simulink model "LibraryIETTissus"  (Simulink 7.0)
settings: Solver=ode45  StartTime=0.0  StopTime=10  RelTol=1e-3
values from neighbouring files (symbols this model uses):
  b = S/Sm    (= 0.1)    [Constantes.m]    (also in ConstantesBck.m)
  beta = 0.95    [Constantes.m]    (also in ResCourV1.m = 1; ResCrV1.m = 1; ResEnerV1.m = 1; ConstantesBck.m)
  C = 1    [Constantes.m]    (also in ConstantesBck.m)
  Cdl = 603E-9    (= 6.03e-07)    [Constantes.m]    (also in ResCourV1.m = 7.313e-07; ResCrV1.m = 7.313e-07; ResEnerV1.m = 7.313e-07; ConstantesBck.m)
  Cmem = 1E-6*Sm*(1-b)    (= 2.826e-08)    [Constantes.m]    (also in ConstantesBck.m = 3.14e-11; ImpedanceZtissus.m = 4e-08; Ztissus.m = 4e-08; CalculCharge.m = 1)
  Fact = 10^2    (= 100)    [Constantes.m]    (also in ConstantesBck.m)
  gk = 36    [Constantes.m]    (also in ConstantesBck.m; sim_hh.m)
  gl = 0.3    [Constantes.m]    (also in ConstantesBck.m; sim_hh.m)
  gna = 120    [Constantes.m]    (also in ConstantesBck.m; sim_hh.m)
  h0 = 0.5961    [Constantes.m]    (also in ConstantesBck.m)
  m0 = 0.0529    [Constantes.m]    (also in ConstantesBck.m)
  mK = 0    [Constantes.m]    (also in ConstantesBck.m)
  mL = 0    [Constantes.m]    (also in ConstantesBck.m)
  mNa = 0    [Constantes.m]    (also in ConstantesBck.m)
  n0 = 0.3177    [Constantes.m]    (also in ConstantesBck.m)
  rapportIE = 10    [Constantes.m]
  Rcan = 6.398E3*Sm*(1-b)    (= 180.80748)    [Constantes.m]    (also in ConstantesBck.m = 0.03454; ImpedanceZtissus.m = 44; Ztissus.m = 44)
  Rct = 185.6E3    (= 185600)    [Constantes.m]    (also in ResCourV1.m = 605200; ResCrV1.m = 605200; ResEnerV1.m = 605200; ConstantesBck.m)
  Rext = 2.9E3    (= 2900)    [Constantes.m]    (also in ConstantesBck.m)
  Rint = 2.9E2    (= 290)    [Constantes.m]    (also in ConstantesBck.m = 400)
  sigma = 66466    [Constantes.m]    (also in ResCourV1.m = 68000; ResCrV1.m = 68000; ResEnerV1.m = 68000; ConstantesBck.m)
  Sm = 3.14e-2    (= 0.0314)    [Constantes.m]    (also in ConstantesBck.m = 0.000314)
  Vk = -82    [Constantes.m]    (also in ConstantesBck.m)
  Vl = -59    [Constantes.m]    (also in ConstantesBck.m)
  Vna = 45    [Constantes.m]    (also in ConstantesBck.m)
  Vr = -70    [Constantes.m]    (also in ConstantesBck.m)
undefined symbols (not defined in the file or in its folder): ln
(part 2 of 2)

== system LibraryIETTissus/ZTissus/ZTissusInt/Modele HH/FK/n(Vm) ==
  note: V
  note: alpha_*(1-n)
  note: beta_n*n
  note: n
  note: n
  Vm : Inport  OutDataType=sfix(16)  OutScaling=2^0
  (1-n) : Fcn  Expr=1-u
  Integrator1 : Integrator  InitialCondition=n0
  Product : Product  OutDataType=sfix(16)  OutScaling=2^0
  Product1 : Product  OutDataType=sfix(16)  OutScaling=2^0
  Sum1 : Sum  Inputs=+-  OutDataType=sfix(16)  OutScaling=2^0
  V : Fcn  Expr=u-Vr
  alpha_n : Fcn  Expr=(0.01*(10-u))/(exp((10-u)/10)-1)
  beta_n : Fcn  Expr=0.125*exp(-u/80)
  n : Outport  OutDataType=sfix(16)  OutScaling=2^0  InitialOutput=0
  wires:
  V/1 -> alpha_n/1, beta_n/1
  alpha_n/1 -> Product/2
  (1-n)/1 -> Product/1
  beta_n/1 -> Product1/1
  Product/1 -> Sum1/1
  Product1/1 -> Sum1/2
  Sum1/1 -> Integrator1/1
  Integrator1/1 -> (1-n)/1, Product1/2, n/1
  Vm/1 -> V/1

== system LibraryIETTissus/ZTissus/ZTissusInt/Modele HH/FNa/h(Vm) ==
  note: h
  note: h
  note: beta_h*h
  note: alpha_h*(1-h)
  note: V
  Vm : Inport  OutDataType=sfix(16)  OutScaling=2^0
  (1-h) : Fcn  Expr=1-u
  Integrator1 : Integrator  InitialCondition=h0
  Product : Product  OutDataType=sfix(16)  OutScaling=2^0
  Product1 : Product  OutDataType=sfix(16)  OutScaling=2^0
  Sum1 : Sum  Inputs=+-  OutDataType=sfix(16)  OutScaling=2^0
  V : Fcn  Expr=u-Vr
  alpha_h : Fcn  Expr=0.07*exp(-u/20)
  beta_h : Fcn  Expr=1/(exp((30-u)/10)+1)
  h : Outport  OutDataType=sfix(16)  OutScaling=2^0  InitialOutput=0
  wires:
  Vm/1 -> V/1
  Integrator1/1 -> h/1, Product1/2, (1-h)/1
  Sum1/1 -> Integrator1/1
  Product1/1 -> Sum1/2
  Product/1 -> Sum1/1
  beta_h/1 -> Product1/1
  (1-h)/1 -> Product/1
  alpha_h/1 -> Product/2
  V/1 -> beta_h/1, alpha_h/1

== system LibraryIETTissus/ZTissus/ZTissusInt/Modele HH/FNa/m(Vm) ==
  note: m
  note: m
  note: beta_m*m
  note: alpha_m*(1-m)
  note: V
  Vm : Inport  OutDataType=sfix(16)  OutScaling=2^0
  (1-m) : Fcn  Expr=1-u
  Integrator1 : Integrator  InitialCondition=m0
  Product : Product  OutDataType=sfix(16)  OutScaling=2^0
  Product1 : Product  OutDataType=sfix(16)  OutScaling=2^0
  Sum1 : Sum  Inputs=+-  OutDataType=sfix(16)  OutScaling=2^0
  V : Fcn  Expr=u-Vr
  alpha_m : Fcn  Expr=(0.1*(25-u))/(exp((25-u)/10)-1)
  beta_m : Fcn  Expr=4*exp(-u/18)
  n : Outport  OutDataType=sfix(16)  OutScaling=2^0  InitialOutput=0
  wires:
  Vm/1 -> V/1
  Integrator1/1 -> n/1, Product1/2, (1-m)/1
  Sum1/1 -> Integrator1/1
  Product1/1 -> Sum1/2
  Product/1 -> Sum1/1
  beta_m/1 -> Product1/1
  (1-m)/1 -> Product/1
  alpha_m/1 -> Product/2
  V/1 -> beta_m/1, alpha_m/1

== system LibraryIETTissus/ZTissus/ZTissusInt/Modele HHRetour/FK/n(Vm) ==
  note: V
  note: alpha_*(1-n)
  note: beta_n*n
  note: n
  note: n
  Vm : Inport  OutDataType=sfix(16)  OutScaling=2^0
  (1-n) : Fcn  Expr=1-u
  Integrator1 : Integrator  InitialCondition=n0
  Product : Product  OutDataType=sfix(16)  OutScaling=2^0
  Product1 : Product  OutDataType=sfix(16)  OutScaling=2^0
  Sum1 : Sum  Inputs=+-  OutDataType=sfix(16)  OutScaling=2^0
  V : Fcn  Expr=u-Vr
  alpha_n : Fcn  Expr=(0.01*(10-u))/(exp((10-u)/10)-1)
  beta_n : Fcn  Expr=0.125*exp(-u/80)
  n : Outport  OutDataType=sfix(16)  OutScaling=2^0  InitialOutput=0
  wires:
  V/1 -> alpha_n/1, beta_n/1
  alpha_n/1 -> Product/2
  (1-n)/1 -> Product/1
  beta_n/1 -> Product1/1
  Product/1 -> Sum1/1
  Product1/1 -> Sum1/2
  Sum1/1 -> Integrator1/1
  Integrator1/1 -> (1-n)/1, Product1/2, n/1
  Vm/1 -> V/1

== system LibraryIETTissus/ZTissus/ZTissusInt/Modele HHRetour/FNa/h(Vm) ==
  note: h
  note: h
  note: beta_h*h
  note: alpha_h*(1-h)
  note: V
  Vm : Inport  OutDataType=sfix(16)  OutScaling=2^0
  (1-h) : Fcn  Expr=1-u
  Integrator1 : Integrator  InitialCondition=h0
  Product : Product  OutDataType=sfix(16)  OutScaling=2^0
  Product1 : Product  OutDataType=sfix(16)  OutScaling=2^0
  Sum1 : Sum  Inputs=+-  OutDataType=sfix(16)  OutScaling=2^0
  V : Fcn  Expr=u-Vr
  alpha_h : Fcn  Expr=0.07*exp(-u/20)
  beta_h : Fcn  Expr=1/(exp((30-u)/10)+1)
  h : Outport  OutDataType=sfix(16)  OutScaling=2^0  InitialOutput=0
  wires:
  Vm/1 -> V/1
  Integrator1/1 -> h/1, Product1/2, (1-h)/1
  Sum1/1 -> Integrator1/1
  Product1/1 -> Sum1/2
  Product/1 -> Sum1/1
  beta_h/1 -> Product1/1
  (1-h)/1 -> Product/1
  alpha_h/1 -> Product/2
  V/1 -> beta_h/1, alpha_h/1

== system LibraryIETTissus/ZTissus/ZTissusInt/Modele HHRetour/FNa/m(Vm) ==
  note: m
  note: m
  note: beta_m*m
  note: alpha_m*(1-m)
  note: V
  Vm : Inport  OutDataType=sfix(16)  OutScaling=2^0
  (1-m) : Fcn  Expr=1-u
  Integrator1 : Integrator  InitialCondition=m0
  Product : Product  OutDataType=sfix(16)  OutScaling=2^0
  Product1 : Product  OutDataType=sfix(16)  OutScaling=2^0
  Sum1 : Sum  Inputs=+-  OutDataType=sfix(16)  OutScaling=2^0
  V : Fcn  Expr=u-Vr
  alpha_m : Fcn  Expr=(0.1*(25-u))/(exp((25-u)/10)-1)
  beta_m : Fcn  Expr=4*exp(-u/18)
  n : Outport  OutDataType=sfix(16)  OutScaling=2^0  InitialOutput=0
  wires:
  Vm/1 -> V/1
  Integrator1/1 -> n/1, Product1/2, (1-m)/1
  Sum1/1 -> Integrator1/1
  Product1/1 -> Sum1/2
  Product/1 -> Sum1/1
  beta_m/1 -> Product1/1
  (1-m)/1 -> Product/1
  alpha_m/1 -> Product/2
  V/1 -> beta_m/1, alpha_m/1

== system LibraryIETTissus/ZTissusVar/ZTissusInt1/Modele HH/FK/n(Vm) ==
  note: V
  note: alpha_*(1-n)
  note: beta_n*n
  note: n
  note: n
  Vm : Inport  OutDataType=sfix(16)  OutScaling=2^0
  (1-n) : Fcn  Expr=1-u
  Integrator1 : Integrator  InitialCondition=n0
  Product : Product  OutDataType=sfix(16)  OutScaling=2^0
  Product1 : Product  OutDataType=sfix(16)  OutScaling=2^0
  Sum1 : Sum  Inputs=+-  OutDataType=sfix(16)  OutScaling=2^0
  V : Fcn  Expr=u-Vr
  alpha_n : Fcn  Expr=(0.01*(10-u))/(exp((10-u)/10)-1)
  beta_n : Fcn  Expr=0.125*exp(-u/80)
  n : Outport  OutDataType=sfix(16)  OutScaling=2^0  InitialOutput=0
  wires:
  V/1 -> alpha_n/1, beta_n/1
  alpha_n/1 -> Product/2
  (1-n)/1 -> Product/1
  beta_n/1 -> Product1/1
  Product/1 -> Sum1/1
  Product1/1 -> Sum1/2
  Sum1/1 -> Integrator1/1
  Integrator1/1 -> (1-n)/1, Product1/2, n/1
  Vm/1 -> V/1

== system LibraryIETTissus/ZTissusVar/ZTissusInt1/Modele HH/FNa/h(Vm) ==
  note: h
  note: h
  note: beta_h*h
  note: alpha_h*(1-h)
  note: V
  Vm : Inport  OutDataType=sfix(16)  OutScaling=2^0
  (1-h) : Fcn  Expr=1-u
  Integrator1 : Integrator  InitialCondition=h0
  Product : Product  OutDataType=sfix(16)  OutScaling=2^0
  Product1 : Product  OutDataType=sfix(16)  OutScaling=2^0
  Sum1 : Sum  Inputs=+-  OutDataType=sfix(16)  OutScaling=2^0
  V : Fcn  Expr=u-Vr
  alpha_h : Fcn  Expr=0.07*exp(-u/20)
  beta_h : Fcn  Expr=1/(exp((30-u)/10)+1)
  h : Outport  OutDataType=sfix(16)  OutScaling=2^0  InitialOutput=0
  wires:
  Vm/1 -> V/1
  Integrator1/1 -> h/1, Product1/2, (1-h)/1
  Sum1/1 -> Integrator1/1
  Product1/1 -> Sum1/2
  Product/1 -> Sum1/1
  beta_h/1 -> Product1/1
  (1-h)/1 -> Product/1
  alpha_h/1 -> Product/2
  V/1 -> beta_h/1, alpha_h/1

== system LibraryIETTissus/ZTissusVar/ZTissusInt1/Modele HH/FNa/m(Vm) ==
  note: m
  note: m
  note: beta_m*m
  note: alpha_m*(1-m)
  note: V
  Vm : Inport  OutDataType=sfix(16)  OutScaling=2^0
  (1-m) : Fcn  Expr=1-u
  Integrator1 : Integrator  InitialCondition=m0
  Product : Product  OutDataType=sfix(16)  OutScaling=2^0
  Product1 : Product  OutDataType=sfix(16)  OutScaling=2^0
  Sum1 : Sum  Inputs=+-  OutDataType=sfix(16)  OutScaling=2^0
  V : Fcn  Expr=u-Vr
  alpha_m : Fcn  Expr=(0.1*(25-u))/(exp((25-u)/10)-1)
  beta_m : Fcn  Expr=4*exp(-u/18)
  n : Outport  OutDataType=sfix(16)  OutScaling=2^0  InitialOutput=0
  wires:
  Vm/1 -> V/1
  Integrator1/1 -> n/1, Product1/2, (1-m)/1
  Sum1/1 -> Integrator1/1
  Product1/1 -> Sum1/2
  Product/1 -> Sum1/1
  beta_m/1 -> Product1/1
  (1-m)/1 -> Product/1
  alpha_m/1 -> Product/2
  V/1 -> beta_m/1, alpha_m/1

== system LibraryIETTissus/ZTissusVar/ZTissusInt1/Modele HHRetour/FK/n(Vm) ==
  note: V
  note: alpha_*(1-n)
  note: beta_n*n
  note: n
  note: n
  Vm : Inport  OutDataType=sfix(16)  OutScaling=2^0
  (1-n) : Fcn  Expr=1-u
  Integrator1 : Integrator  InitialCondition=n0
  Product : Product  OutDataType=sfix(16)  OutScaling=2^0
  Product1 : Product  OutDataType=sfix(16)  OutScaling=2^0
  Sum1 : Sum  Inputs=+-  OutDataType=sfix(16)  OutScaling=2^0
  V : Fcn  Expr=u-Vr
  alpha_n : Fcn  Expr=(0.01*(10-u))/(exp((10-u)/10)-1)
  beta_n : Fcn  Expr=0.125*exp(-u/80)
  n : Outport  OutDataType=sfix(16)  OutScaling=2^0  InitialOutput=0
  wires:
  V/1 -> alpha_n/1, beta_n/1
  alpha_n/1 -> Product/2
  (1-n)/1 -> Product/1
  beta_n/1 -> Product1/1
  Product/1 -> Sum1/1
  Product1/1 -> Sum1/2
  Sum1/1 -> Integrator1/1
  Integrator1/1 -> (1-n)/1, Product1/2, n/1
  Vm/1 -> V/1

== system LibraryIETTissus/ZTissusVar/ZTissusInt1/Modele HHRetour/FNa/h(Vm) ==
  note: h
  note: h
  note: beta_h*h
  note: alpha_h*(1-h)
  note: V
  Vm : Inport  OutDataType=sfix(16)  OutScaling=2^0
  (1-h) : Fcn  Expr=1-u
  Integrator1 : Integrator  InitialCondition=h0
  Product : Product  OutDataType=sfix(16)  OutScaling=2^0
  Product1 : Product  OutDataType=sfix(16)  OutScaling=2^0
  Sum1 : Sum  Inputs=+-  OutDataType=sfix(16)  OutScaling=2^0
  V : Fcn  Expr=u-Vr
  alpha_h : Fcn  Expr=0.07*exp(-u/20)
  beta_h : Fcn  Expr=1/(exp((30-u)/10)+1)
  h : Outport  OutDataType=sfix(16)  OutScaling=2^0  InitialOutput=0
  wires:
  Vm/1 -> V/1
  Integrator1/1 -> h/1, Product1/2, (1-h)/1
  Sum1/1 -> Integrator1/1
  Product1/1 -> Sum1/2
  Product/1 -> Sum1/1
  beta_h/1 -> Product1/1
  (1-h)/1 -> Product/1
  alpha_h/1 -> Product/2
  V/1 -> beta_h/1, alpha_h/1

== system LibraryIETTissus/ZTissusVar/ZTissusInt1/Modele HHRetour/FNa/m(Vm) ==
  note: m
  note: m
  note: beta_m*m
  note: alpha_m*(1-m)
  note: V
  Vm : Inport  OutDataType=sfix(16)  OutScaling=2^0
  (1-m) : Fcn  Expr=1-u
  Integrator1 : Integrator  InitialCondition=m0
  Product : Product  OutDataType=sfix(16)  OutScaling=2^0
  Product1 : Product  OutDataType=sfix(16)  OutScaling=2^0
  Sum1 : Sum  Inputs=+-  OutDataType=sfix(16)  OutScaling=2^0
  V : Fcn  Expr=u-Vr
  alpha_m : Fcn  Expr=(0.1*(25-u))/(exp((25-u)/10)-1)
  beta_m : Fcn  Expr=4*exp(-u/18)
  n : Outport  OutDataType=sfix(16)  OutScaling=2^0  InitialOutput=0
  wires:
  Vm/1 -> V/1
  Integrator1/1 -> n/1, Product1/2, (1-m)/1
  Sum1/1 -> Integrator1/1
  Product1/1 -> Sum1/2
  Product/1 -> Sum1/1
  beta_m/1 -> Product1/1
  (1-m)/1 -> Product/1
  alpha_m/1 -> Product/2
  V/1 -> beta_m/1, alpha_m/1

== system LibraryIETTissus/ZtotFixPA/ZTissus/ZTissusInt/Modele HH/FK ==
  note: gkm
  note: (Vm-Vk0)
  FKIn : Inport  OutDataType=sfix(16)  OutScaling=2^0
  (Vm-Vk0) : Fcn  Expr=(u-Vk)
  Product : Product  OutDataType=sfix(16)  OutScaling=2^0
  n(Vm) : Subsystem
  n^4 : Fcn  Expr=gk*(u^4)
  FKout : Outport  OutDataType=sfix(16)  OutScaling=2^0  InitialOutput=0
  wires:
  n(Vm)/1(n) -> n^4/1
  (Vm-Vk0)/1 -> Product/2
  Product/1 -> FKout/1
  n^4/1 -> Product/1
  FKIn/1 -> n(Vm)/1(Vm), (Vm-Vk0)/1

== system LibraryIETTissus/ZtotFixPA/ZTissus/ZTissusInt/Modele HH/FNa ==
  note: gNa*m^3
  note: m
  note: h
  note: gNam
  note: (Vm-VNa0)
  FNaIn : Inport  OutDataType=sfix(16)  OutScaling=2^0
  (Vm-VNa0) : Fcn  Expr=(u-Vna)
  Product : Product  OutDataType=sfix(16)  OutScaling=2^0
  Product1 : Product  OutDataType=sfix(16)  OutScaling=2^0
  gna*m^3 : Fcn  Expr=gna*u^3
  h(Vm) : Subsystem
  m(Vm) : Subsystem
  FNaOut : Outport  OutDataType=sfix(16)  OutScaling=2^0  InitialOutput=0
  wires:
  (Vm-VNa0)/1 -> Product1/2
  gna*m^3/1 -> Product/1
  Product1/1 -> FNaOut/1
  FNaIn/1 -> m(Vm)/1(Vm), h(Vm)/1(Vm), (Vm-VNa0)/1
  m(Vm)/1(n) -> gna*m^3/1
  h(Vm)/1(h) -> Product/2
  Product/1 -> Product1/1

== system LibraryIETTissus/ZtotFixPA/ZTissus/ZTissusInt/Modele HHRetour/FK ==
  note: gkm
  note: (Vm-Vk0)
  FKIn : Inport  OutDataType=sfix(16)  OutScaling=2^0
  (Vm-Vk0) : Fcn  Expr=(u-Vk)
  Product : Product  OutDataType=sfix(16)  OutScaling=2^0
  n(Vm) : Subsystem
  n^4 : Fcn  Expr=gk*(u^4)
  FKout : Outport  OutDataType=sfix(16)  OutScaling=2^0  InitialOutput=0
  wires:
  n(Vm)/1(n) -> n^4/1
  (Vm-Vk0)/1 -> Product/2
  Product/1 -> FKout/1
  n^4/1 -> Product/1
  FKIn/1 -> n(Vm)/1(Vm), (Vm-Vk0)/1

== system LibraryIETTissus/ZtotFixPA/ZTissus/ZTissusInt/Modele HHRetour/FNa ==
  note: gNa*m^3
  note: m
  note: h
  note: gNam
  note: (Vm-VNa0)
  FNaIn : Inport  OutDataType=sfix(16)  OutScaling=2^0
  (Vm-VNa0) : Fcn  Expr=(u-Vna)
  Product : Product  OutDataType=sfix(16)  OutScaling=2^0
  Product1 : Product  OutDataType=sfix(16)  OutScaling=2^0
  gna*m^3 : Fcn  Expr=gna*u^3
  h(Vm) : Subsystem
  m(Vm) : Subsystem
  FNaOut : Outport  OutDataType=sfix(16)  OutScaling=2^0  InitialOutput=0
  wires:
  (Vm-VNa0)/1 -> Product1/2
  gna*m^3/1 -> Product/1
  Product1/1 -> FNaOut/1
  FNaIn/1 -> m(Vm)/1(Vm), h(Vm)/1(Vm), (Vm-VNa0)/1
  m(Vm)/1(n) -> gna*m^3/1
  h(Vm)/1(h) -> Product/2
  Product/1 -> Product1/1

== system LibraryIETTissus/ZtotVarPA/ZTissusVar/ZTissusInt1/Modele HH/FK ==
  note: gkm
  note: (Vm-Vk0)
  FKIn : Inport  OutDataType=sfix(16)  OutScaling=2^0
  (Vm-Vk0) : Fcn  Expr=(u-Vk)
  Product : Product  OutDataType=sfix(16)  OutScaling=2^0
  n(Vm) : Subsystem
  n^4 : Fcn  Expr=gk*(u^4)
  FKout : Outport  OutDataType=sfix(16)  OutScaling=2^0  InitialOutput=0
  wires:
  n(Vm)/1(n) -> n^4/1
  (Vm-Vk0)/1 -> Product/2
  Product/1 -> FKout/1
  n^4/1 -> Product/1
  FKIn/1 -> n(Vm)/1(Vm), (Vm-Vk0)/1

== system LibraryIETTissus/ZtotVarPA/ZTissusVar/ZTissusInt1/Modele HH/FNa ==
  note: gNa*m^3
  note: m
  note: h
  note: gNam
  note: (Vm-VNa0)
  FNaIn : Inport  OutDataType=sfix(16)  OutScaling=2^0
  (Vm-VNa0) : Fcn  Expr=(u-Vna)
  Product : Product  OutDataType=sfix(16)  OutScaling=2^0
  Product1 : Product  OutDataType=sfix(16)  OutScaling=2^0
  gna*m^3 : Fcn  Expr=gna*u^3
  h(Vm) : Subsystem
  m(Vm) : Subsystem
  FNaOut : Outport  OutDataType=sfix(16)  OutScaling=2^0  InitialOutput=0
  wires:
  (Vm-VNa0)/1 -> Product1/2
  gna*m^3/1 -> Product/1
  Product1/1 -> FNaOut/1
  FNaIn/1 -> m(Vm)/1(Vm), h(Vm)/1(Vm), (Vm-VNa0)/1
  m(Vm)/1(n) -> gna*m^3/1
  h(Vm)/1(h) -> Product/2
  Product/1 -> Product1/1

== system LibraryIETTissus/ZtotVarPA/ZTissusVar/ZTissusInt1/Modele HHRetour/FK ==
  note: gkm
  note: (Vm-Vk0)
  FKIn : Inport  OutDataType=sfix(16)  OutScaling=2^0
  (Vm-Vk0) : Fcn  Expr=(u-Vk)
  Product : Product  OutDataType=sfix(16)  OutScaling=2^0
  n(Vm) : Subsystem
  n^4 : Fcn  Expr=gk*(u^4)
  FKout : Outport  OutDataType=sfix(16)  OutScaling=2^0  InitialOutput=0
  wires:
  n(Vm)/1(n) -> n^4/1
  (Vm-Vk0)/1 -> Product/2
  Product/1 -> FKout/1
  n^4/1 -> Product/1
  FKIn/1 -> n(Vm)/1(Vm), (Vm-Vk0)/1

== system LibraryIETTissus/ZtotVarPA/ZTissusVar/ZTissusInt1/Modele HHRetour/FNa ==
  note: gNa*m^3
  note: m
  note: h
  note: gNam
  note: (Vm-VNa0)
  FNaIn : Inport  OutDataType=sfix(16)  OutScaling=2^0
  (Vm-VNa0) : Fcn  Expr=(u-Vna)
  Product : Product  OutDataType=sfix(16)  OutScaling=2^0
  Product1 : Product  OutDataType=sfix(16)  OutScaling=2^0
  gna*m^3 : Fcn  Expr=gna*u^3
  h(Vm) : Subsystem
  m(Vm) : Subsystem
  FNaOut : Outport  OutDataType=sfix(16)  OutScaling=2^0  InitialOutput=0
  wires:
  (Vm-VNa0)/1 -> Product1/2
  gna*m^3/1 -> Product/1
  Product1/1 -> FNaOut/1
  FNaIn/1 -> m(Vm)/1(Vm), h(Vm)/1(Vm), (Vm-VNa0)/1
  m(Vm)/1(n) -> gna*m^3/1
  h(Vm)/1(h) -> Product/2
  Product/1 -> Product1/1

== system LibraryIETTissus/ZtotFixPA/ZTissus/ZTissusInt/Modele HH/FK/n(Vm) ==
  note: V
  note: alpha_*(1-n)
  note: beta_n*n
  note: n
  note: n
  Vm : Inport  OutDataType=sfix(16)  OutScaling=2^0
  (1-n) : Fcn  Expr=1-u
  Integrator1 : Integrator  InitialCondition=n0
  Product : Product  OutDataType=sfix(16)  OutScaling=2^0
  Product1 : Product  OutDataType=sfix(16)  OutScaling=2^0
  Sum1 : Sum  Inputs=+-  OutDataType=sfix(16)  OutScaling=2^0
  V : Fcn  Expr=u-Vr
  alpha_n : Fcn  Expr=(0.01*(10-u))/(exp((10-u)/10)-1)
  beta_n : Fcn  Expr=0.125*exp(-u/80)
  n : Outport  OutDataType=sfix(16)  OutScaling=2^0  InitialOutput=0
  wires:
  V/1 -> alpha_n/1, beta_n/1
  alpha_n/1 -> Product/2
  (1-n)/1 -> Product/1
  beta_n/1 -> Product1/1
  Product/1 -> Sum1/1
  Product1/1 -> Sum1/2
  Sum1/1 -> Integrator1/1
  Integrator1/1 -> (1-n)/1, Product1/2, n/1
  Vm/1 -> V/1

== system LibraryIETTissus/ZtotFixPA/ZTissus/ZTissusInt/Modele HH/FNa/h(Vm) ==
  note: h
  note: h
  note: beta_h*h
  note: alpha_h*(1-h)
  note: V
  Vm : Inport  OutDataType=sfix(16)  OutScaling=2^0
  (1-h) : Fcn  Expr=1-u
  Integrator1 : Integrator  InitialCondition=h0
  Product : Product  OutDataType=sfix(16)  OutScaling=2^0
  Product1 : Product  OutDataType=sfix(16)  OutScaling=2^0
  Sum1 : Sum  Inputs=+-  OutDataType=sfix(16)  OutScaling=2^0
  V : Fcn  Expr=u-Vr
  alpha_h : Fcn  Expr=0.07*exp(-u/20)
  beta_h : Fcn  Expr=1/(exp((30-u)/10)+1)
  h : Outport  OutDataType=sfix(16)  OutScaling=2^0  InitialOutput=0
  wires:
  Vm/1 -> V/1
  Integrator1/1 -> h/1, Product1/2, (1-h)/1
  Sum1/1 -> Integrator1/1
  Product1/1 -> Sum1/2
  Product/1 -> Sum1/1
  beta_h/1 -> Product1/1
  (1-h)/1 -> Product/1
  alpha_h/1 -> Product/2
  V/1 -> beta_h/1, alpha_h/1

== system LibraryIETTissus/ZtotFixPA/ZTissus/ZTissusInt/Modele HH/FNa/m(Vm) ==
  note: m
  note: m
  note: beta_m*m
  note: alpha_m*(1-m)
  note: V
  Vm : Inport  OutDataType=sfix(16)  OutScaling=2^0
  (1-m) : Fcn  Expr=1-u
  Integrator1 : Integrator  InitialCondition=m0
  Product : Product  OutDataType=sfix(16)  OutScaling=2^0
  Product1 : Product  OutDataType=sfix(16)  OutScaling=2^0
  Sum1 : Sum  Inputs=+-  OutDataType=sfix(16)  OutScaling=2^0
  V : Fcn  Expr=u-Vr
  alpha_m : Fcn  Expr=(0.1*(25-u))/(exp((25-u)/10)-1)
  beta_m : Fcn  Expr=4*exp(-u/18)
  n : Outport  OutDataType=sfix(16)  OutScaling=2^0  InitialOutput=0
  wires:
  Vm/1 -> V/1
  Integrator1/1 -> n/1, Product1/2, (1-m)/1
  Sum1/1 -> Integrator1/1
  Product1/1 -> Sum1/2
  Product/1 -> Sum1/1
  beta_m/1 -> Product1/1
  (1-m)/1 -> Product/1
  alpha_m/1 -> Product/2
  V/1 -> beta_m/1, alpha_m/1

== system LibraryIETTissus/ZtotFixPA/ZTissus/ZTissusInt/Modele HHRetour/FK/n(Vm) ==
  note: V
  note: alpha_*(1-n)
  note: beta_n*n
  note: n
  note: n
  Vm : Inport  OutDataType=sfix(16)  OutScaling=2^0
  (1-n) : Fcn  Expr=1-u
  Integrator1 : Integrator  InitialCondition=n0
  Product : Product  OutDataType=sfix(16)  OutScaling=2^0
  Product1 : Product  OutDataType=sfix(16)  OutScaling=2^0
  Sum1 : Sum  Inputs=+-  OutDataType=sfix(16)  OutScaling=2^0
  V : Fcn  Expr=u-Vr
  alpha_n : Fcn  Expr=(0.01*(10-u))/(exp((10-u)/10)-1)
  beta_n : Fcn  Expr=0.125*exp(-u/80)
  n : Outport  OutDataType=sfix(16)  OutScaling=2^0  InitialOutput=0
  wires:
  V/1 -> alpha_n/1, beta_n/1
  alpha_n/1 -> Product/2
  (1-n)/1 -> Product/1
  beta_n/1 -> Product1/1
  Product/1 -> Sum1/1
  Product1/1 -> Sum1/2
  Sum1/1 -> Integrator1/1
  Integrator1/1 -> (1-n)/1, Product1/2, n/1
  Vm/1 -> V/1

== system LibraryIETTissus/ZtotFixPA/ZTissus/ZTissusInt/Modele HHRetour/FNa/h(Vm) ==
  note: h
  note: h
  note: beta_h*h
  note: alpha_h*(1-h)
  note: V
  Vm : Inport  OutDataType=sfix(16)  OutScaling=2^0
  (1-h) : Fcn  Expr=1-u
  Integrator1 : Integrator  InitialCondition=h0
  Product : Product  OutDataType=sfix(16)  OutScaling=2^0
  Product1 : Product  OutDataType=sfix(16)  OutScaling=2^0
  Sum1 : Sum  Inputs=+-  OutDataType=sfix(16)  OutScaling=2^0
  V : Fcn  Expr=u-Vr
  alpha_h : Fcn  Expr=0.07*exp(-u/20)
  beta_h : Fcn  Expr=1/(exp((30-u)/10)+1)
  h : Outport  OutDataType=sfix(16)  OutScaling=2^0  InitialOutput=0
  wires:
  Vm/1 -> V/1
  Integrator1/1 -> h/1, Product1/2, (1-h)/1
  Sum1/1 -> Integrator1/1
  Product1/1 -> Sum1/2
  Product/1 -> Sum1/1
  beta_h/1 -> Product1/1
  (1-h)/1 -> Product/1
  alpha_h/1 -> Product/2
  V/1 -> beta_h/1, alpha_h/1

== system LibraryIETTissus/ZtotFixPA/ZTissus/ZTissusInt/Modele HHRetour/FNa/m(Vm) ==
  note: m
  note: m
  note: beta_m*m
  note: alpha_m*(1-m)
  note: V
  Vm : Inport  OutDataType=sfix(16)  OutScaling=2^0
  (1-m) : Fcn  Expr=1-u
  Integrator1 : Integrator  InitialCondition=m0
  Product : Product  OutDataType=sfix(16)  OutScaling=2^0
  Product1 : Product  OutDataType=sfix(16)  OutScaling=2^0
  Sum1 : Sum  Inputs=+-  OutDataType=sfix(16)  OutScaling=2^0
  V : Fcn  Expr=u-Vr
  alpha_m : Fcn  Expr=(0.1*(25-u))/(exp((25-u)/10)-1)
  beta_m : Fcn  Expr=4*exp(-u/18)
  n : Outport  OutDataType=sfix(16)  OutScaling=2^0  InitialOutput=0
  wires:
  Vm/1 -> V/1
  Integrator1/1 -> n/1, Product1/2, (1-m)/1
  Sum1/1 -> Integrator1/1
  Product1/1 -> Sum1/2
  Product/1 -> Sum1/1
  beta_m/1 -> Product1/1
  (1-m)/1 -> Product/1
  alpha_m/1 -> Product/2
  V/1 -> beta_m/1, alpha_m/1

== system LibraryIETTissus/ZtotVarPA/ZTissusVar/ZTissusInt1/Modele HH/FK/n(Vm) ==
  note: V
  note: alpha_*(1-n)
  note: beta_n*n
  note: n
  note: n
  Vm : Inport  OutDataType=sfix(16)  OutScaling=2^0
  (1-n) : Fcn  Expr=1-u
  Integrator1 : Integrator  InitialCondition=n0
  Product : Product  OutDataType=sfix(16)  OutScaling=2^0
  Product1 : Product  OutDataType=sfix(16)  OutScaling=2^0
  Sum1 : Sum  Inputs=+-  OutDataType=sfix(16)  OutScaling=2^0
  V : Fcn  Expr=u-Vr
  alpha_n : Fcn  Expr=(0.01*(10-u))/(exp((10-u)/10)-1)
  beta_n : Fcn  Expr=0.125*exp(-u/80)
  n : Outport  OutDataType=sfix(16)  OutScaling=2^0  InitialOutput=0
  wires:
  V/1 -> alpha_n/1, beta_n/1
  alpha_n/1 -> Product/2
  (1-n)/1 -> Product/1
  beta_n/1 -> Product1/1
  Product/1 -> Sum1/1
  Product1/1 -> Sum1/2
  Sum1/1 -> Integrator1/1
  Integrator1/1 -> (1-n)/1, Product1/2, n/1
  Vm/1 -> V/1

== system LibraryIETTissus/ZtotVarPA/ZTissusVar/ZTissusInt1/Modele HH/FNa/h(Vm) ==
  note: h
  note: h
  note: beta_h*h
  note: alpha_h*(1-h)
  note: V
  Vm : Inport  OutDataType=sfix(16)  OutScaling=2^0
  (1-h) : Fcn  Expr=1-u
  Integrator1 : Integrator  InitialCondition=h0
  Product : Product  OutDataType=sfix(16)  OutScaling=2^0
  Product1 : Product  OutDataType=sfix(16)  OutScaling=2^0
  Sum1 : Sum  Inputs=+-  OutDataType=sfix(16)  OutScaling=2^0
  V : Fcn  Expr=u-Vr
  alpha_h : Fcn  Expr=0.07*exp(-u/20)
  beta_h : Fcn  Expr=1/(exp((30-u)/10)+1)
  h : Outport  OutDataType=sfix(16)  OutScaling=2^0  InitialOutput=0
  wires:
  Vm/1 -> V/1
  Integrator1/1 -> h/1, Product1/2, (1-h)/1
  Sum1/1 -> Integrator1/1
  Product1/1 -> Sum1/2
  Product/1 -> Sum1/1
  beta_h/1 -> Product1/1
  (1-h)/1 -> Product/1
  alpha_h/1 -> Product/2
  V/1 -> beta_h/1, alpha_h/1

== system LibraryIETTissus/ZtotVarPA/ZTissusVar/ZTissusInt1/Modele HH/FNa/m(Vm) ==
  note: m
  note: m
  note: beta_m*m
  note: alpha_m*(1-m)
  note: V
  Vm : Inport  OutDataType=sfix(16)  OutScaling=2^0
  (1-m) : Fcn  Expr=1-u
  Integrator1 : Integrator  InitialCondition=m0
  Product : Product  OutDataType=sfix(16)  OutScaling=2^0
  Product1 : Product  OutDataType=sfix(16)  OutScaling=2^0
  Sum1 : Sum  Inputs=+-  OutDataType=sfix(16)  OutScaling=2^0
  V : Fcn  Expr=u-Vr
  alpha_m : Fcn  Expr=(0.1*(25-u))/(exp((25-u)/10)-1)
  beta_m : Fcn  Expr=4*exp(-u/18)
  n : Outport  OutDataType=sfix(16)  OutScaling=2^0  InitialOutput=0
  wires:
  Vm/1 -> V/1
  Integrator1/1 -> n/1, Product1/2, (1-m)/1
  Sum1/1 -> Integrator1/1
  Product1/1 -> Sum1/2
  Product/1 -> Sum1/1
  beta_m/1 -> Product1/1
  (1-m)/1 -> Product/1
  alpha_m/1 -> Product/2
  V/1 -> beta_m/1, alpha_m/1

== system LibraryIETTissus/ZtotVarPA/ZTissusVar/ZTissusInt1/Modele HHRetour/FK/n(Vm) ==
  note: V
  note: alpha_*(1-n)
  note: beta_n*n
  note: n
  note: n
  Vm : Inport  OutDataType=sfix(16)  OutScaling=2^0
  (1-n) : Fcn  Expr=1-u
  Integrator1 : Integrator  InitialCondition=n0
  Product : Product  OutDataType=sfix(16)  OutScaling=2^0
  Product1 : Product  OutDataType=sfix(16)  OutScaling=2^0
  Sum1 : Sum  Inputs=+-  OutDataType=sfix(16)  OutScaling=2^0
  V : Fcn  Expr=u-Vr
  alpha_n : Fcn  Expr=(0.01*(10-u))/(exp((10-u)/10)-1)
  beta_n : Fcn  Expr=0.125*exp(-u/80)
  n : Outport  OutDataType=sfix(16)  OutScaling=2^0  InitialOutput=0
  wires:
  V/1 -> alpha_n/1, beta_n/1
  alpha_n/1 -> Product/2
  (1-n)/1 -> Product/1
  beta_n/1 -> Product1/1
  Product/1 -> Sum1/1
  Product1/1 -> Sum1/2
  Sum1/1 -> Integrator1/1
  Integrator1/1 -> (1-n)/1, Product1/2, n/1
  Vm/1 -> V/1

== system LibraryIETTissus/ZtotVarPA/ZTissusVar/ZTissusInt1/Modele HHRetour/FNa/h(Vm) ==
  note: h
  note: h
  note: beta_h*h
  note: alpha_h*(1-h)
  note: V
  Vm : Inport  OutDataType=sfix(16)  OutScaling=2^0
  (1-h) : Fcn  Expr=1-u
  Integrator1 : Integrator  InitialCondition=h0
  Product : Product  OutDataType=sfix(16)  OutScaling=2^0
  Product1 : Product  OutDataType=sfix(16)  OutScaling=2^0
  Sum1 : Sum  Inputs=+-  OutDataType=sfix(16)  OutScaling=2^0
  V : Fcn  Expr=u-Vr
  alpha_h : Fcn  Expr=0.07*exp(-u/20)
  beta_h : Fcn  Expr=1/(exp((30-u)/10)+1)
  h : Outport  OutDataType=sfix(16)  OutScaling=2^0  InitialOutput=0
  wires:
  Vm/1 -> V/1
  Integrator1/1 -> h/1, Product1/2, (1-h)/1
  Sum1/1 -> Integrator1/1
  Product1/1 -> Sum1/2
  Product/1 -> Sum1/1
  beta_h/1 -> Product1/1
  (1-h)/1 -> Product/1
  alpha_h/1 -> Product/2
  V/1 -> beta_h/1, alpha_h/1

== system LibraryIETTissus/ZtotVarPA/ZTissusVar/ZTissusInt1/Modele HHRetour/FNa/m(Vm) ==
  note: m
  note: m
  note: beta_m*m
  note: alpha_m*(1-m)
  note: V
  Vm : Inport  OutDataType=sfix(16)  OutScaling=2^0
  (1-m) : Fcn  Expr=1-u
  Integrator1 : Integrator  InitialCondition=m0
  Product : Product  OutDataType=sfix(16)  OutScaling=2^0
  Product1 : Product  OutDataType=sfix(16)  OutScaling=2^0
  Sum1 : Sum  Inputs=+-  OutDataType=sfix(16)  OutScaling=2^0
  V : Fcn  Expr=u-Vr
  alpha_m : Fcn  Expr=(0.1*(25-u))/(exp((25-u)/10)-1)
  beta_m : Fcn  Expr=4*exp(-u/18)
  n : Outport  OutDataType=sfix(16)  OutScaling=2^0  InitialOutput=0
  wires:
  Vm/1 -> V/1
  Integrator1/1 -> n/1, Product1/2, (1-m)/1
  Sum1/1 -> Integrator1/1
  Product1/1 -> Sum1/2
  Product/1 -> Sum1/1
  beta_m/1 -> Product1/1
  (1-m)/1 -> Product/1
  alpha_m/1 -> Product/2
  V/1 -> beta_m/1, alpha_m/1

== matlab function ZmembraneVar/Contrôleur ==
function [y,temp] = fcn(u,calc)
% This block supports an embeddable subset of the MATLAB language.
% See the help menu for details. 

if u == 0
    y = 0;
    temp = 1E-6;
else
    y = calc;
    temp = u;
end

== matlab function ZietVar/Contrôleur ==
function [y,temp] = fcn(u,calc)
% This block supports an embeddable subset of the MATLAB language.
% See the help menu for details. 

if u == 0
    y = 0;
    temp = 1E-6;
else
    y = calc;
    temp = u;
end

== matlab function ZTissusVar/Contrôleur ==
function [y,temp] = fcn(u,calc)
% This block supports an embeddable subset of the MATLAB language.
% See the help menu for details. 

if u == 0
    y = 0;
    temp = 1E-6;
else
    y = calc;
    temp = u;
end

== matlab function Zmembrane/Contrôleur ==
function [y,temp] = fcn(u,calc)
% This block supports an embeddable subset of the MATLAB language.
% See the help menu for details. 

if u == 0
    y = 0;
    temp = 1E-6;
else
    y = calc;
    temp = u;
end

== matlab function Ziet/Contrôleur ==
function [y,temp] = fcn(u,calc)
% This block supports an embeddable subset of the MATLAB language.
% See the help menu for details. 

if u == 0
    y = 0;
    temp = 1E-6;
else
    y = calc;
    temp = u;
end

== matlab function ZtotFixNPA
/Ziet/Contrôleur ==
function [y,temp] = fcn(u,calc)
% This block supports an embeddable subset of the MATLAB language.
% See the help menu for details. 

if u == 0
    y = 0;
    temp = 1E-6;
else
    y = calc;
    temp = u;
end

== matlab function ZtotFixNPA
/Zmembrane/Contrôleur ==
function [y,temp] = fcn(u,calc)
% This block supports an embeddable subset of the MATLAB language.
% See the help menu for details. 

if u == 0
    y = 0;
    temp = 1E-6;
else
    y = calc;
    temp = u;
end

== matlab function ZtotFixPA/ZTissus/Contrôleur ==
function [y,temp] = fcn(u,calc)
% This block supports an embeddable subset of the MATLAB language.
% See the help menu for details. 

if u == 0
    y = 0;
    temp = 1E-6;
else
    y = calc;
    temp = u;
end

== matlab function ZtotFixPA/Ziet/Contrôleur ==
function [y,temp] = fcn(u,calc)
% This block supports an embeddable subset of the MATLAB language.
% See the help menu for details. 

if u == 0
    y = 0;
    temp = 1E-6;
else
    y = calc;
    temp = u;
end

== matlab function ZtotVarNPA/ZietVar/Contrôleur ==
function [y,temp] = fcn(u,calc)
% This block supports an embeddable subset of the MATLAB language.
% See the help menu for details. 

if u == 0
    y = 0;
    temp = 1E-6;
else
    y = calc;
    temp = u;
end

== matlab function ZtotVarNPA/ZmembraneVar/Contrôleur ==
function [y,temp] = fcn(u,calc)
% This block supports an embeddable subset of the MATLAB language.
% See the help menu for details. 

if u == 0
    y = 0;
    temp = 1E-6;
else
    y = calc;
    temp = u;
end

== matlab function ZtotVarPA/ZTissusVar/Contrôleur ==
function [y,temp] = fcn(u,calc)
% This block supports an embeddable subset of the MATLAB language.
% See the help menu for details. 

if u == 0
    y = 0;
    temp = 1E-6;
else
    y = calc;
    temp = u;
end

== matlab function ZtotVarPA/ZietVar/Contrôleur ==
function [y,temp] = fcn(u,calc)
% This block supports an embeddable subset of the MATLAB language.
% See the help menu for details. 

if u == 0
    y = 0;
    temp = 1E-6;
else
    y = calc;
    temp = u;
end

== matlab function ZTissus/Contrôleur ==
function [y,temp] = fcn(u,calc)
% This block supports an embeddable subset of the MATLAB language.
% See the help menu for details. 

if u == 0
    y = 0;
    temp = 1E-6;
else
    y = calc;
    temp = u;
end
